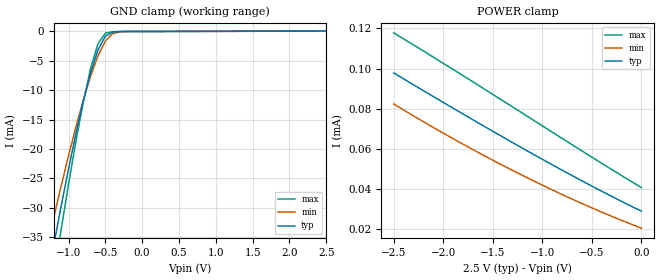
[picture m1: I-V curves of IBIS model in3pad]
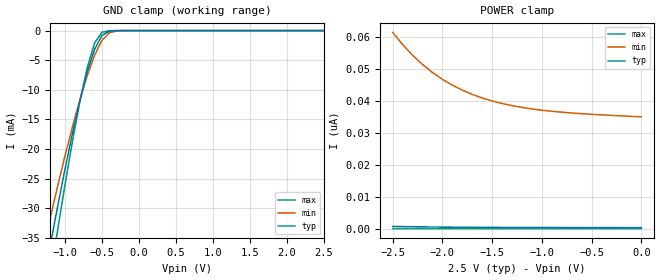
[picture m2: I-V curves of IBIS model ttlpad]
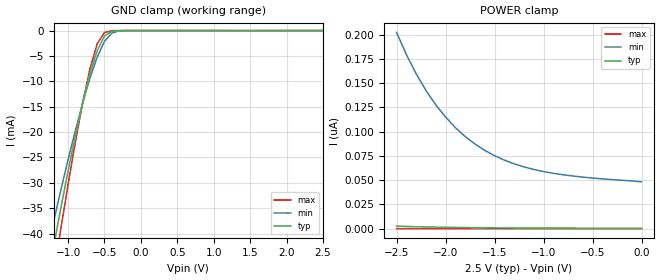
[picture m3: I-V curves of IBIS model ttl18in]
| IBIS file idt45t905z.ibs created by s2ibis2 version 1.2
| North Carolina State University Electronics Research Laboratory  1995
[IBIS ver]   3.2
[File name]   idt45t905z.ibs
[File Rev]   1.0
[Date]   Friday, November 09, 2001
[Source]   Integrated Device Technology, Inc.
[Notes]   Input pins <A> and <AX> can be configured as one of the
   following three models: ttl25in, ttl18in, or hstlin.
   Output pins <Q1> to <Q5> can be configured as one of the
   following three models: ttl25out, ttl18out, or hstlout.
   Please change the column 'model_name' in pin list to select
   the correct model.
[Disclaimer] Integrated Device Technology, Inc. ("IDT") hereby grants the
   user of this IBIS model a non-exclusive, nontransferable
   license to use this IBIS model under the following terms. The
   user is granted this license only to use the IBIS model and is
   not granted rights to sell, copy (except as needed to run the
   IBIS model), rent, lease or sub-license the IBIS model in
   whole or in part, or in modified form to anyone. The User may
   modify the IBIS model to suit its specific applications, but
   rights to derivative works and such modifications shall belong
   to IDT. This IBIS model is provided on an AS IS" basis and IDT
   makes absolutely no warranty with respect to the information
   contained herein. IDT DISCLAIMS AND CUSTOMER WAIVES ALL
   WARRANTIES, EXPRESS AND IMPLIED, INCLUDING WARRANTIES OF
   MERCHANTABILITY AND FITNESS FOR A PARTICULAR PURPOSE. THE
   ENTIRE RISK AS TO QUALITY AND PERFORMANCE IS WITH THE USER
   ACCORDINGLY, IN NO EVENT SHALL IDT BE LIABLE FOR ANY DIRECT OR
   INDIRECT DAMAGES, WHETHER IN CONTRACT OR TORT, INCLUDING ANY
   LOST PROFITS OR OTHER INCIDENTAL, CONSEQUENTIAL, EXEMPLARY, OR
   PUNITIVE DAMAGES ARISING OUT OF THE USE OR APPLICATION OF THE
   IBIS model. Further, IDT reserves the right to make changes
   without notice to any product herein to improve reliability,
   function, or design. IDT does not convey any license under
   patent rights or any other intellectual property rights,
   including those of third parties. IDT is not obligated to
   provide maintenance or support for the licensed IBIS model.
[Copyright]   Copyright 2001, Integrated Device Technology, Inc. all rights
   reserved
|   Component idt45t905z
[Component]   idt45t905z
[Manufacturer]   Integrated Device Technology
|Package   PG28
[Package]
| variable   typ   min   max
R_pkg   2.40000m   2.40000m   2.40000m
L_pkg   0.90000nH   0.90000nH   0.90000nH
C_pkg   60.0000fF   60.0000fF   60.0000fF
[Pin]  signal_name   model_name   R_pin   L_pin   C_pin
1   GL   ttlpad
2   VDD   POWER
3   GND   GND
4   GX   ttlpad
5   VDDQ   POWER
6   Q1   ttl25out
7   AX   ttl25in
8   A   ttl25in
9   Q5   ttl25out
10   VDDQ   POWER
11   GND   GND
12   VDD   POWER
13   VDD   POWER
14   RxS   in3pad
15   TxS   in3pad
16   VDDQ   POWER
17   GND   GND
18   GND   GND
19   VDDQ   POWER
20   Q4   ttl25out
21   Q3   ttl25out
22   GND   GND
23   Q2   ttl25out
24   VDDQ   POWER
25   GND   GND
26   GND   GND
27   VDDQ   POWER
28   GND   GND
[Pin Mapping]  pulldown_ref   pullup_ref   gnd_clamp_ref   power_clamp_ref
1   GND   VDD
2   NC   VDD
3   GND   NC
4   GND   VDD
5   NC   VDDQ
6   GND   VDDQ
7   GND   VDD
8   GND   VDD
9   GND   VDDQ
10   NC   VDDQ
11   GND   NC
12   NC   VDD
13   NC   VDD
14   GND   VDD
15   GND   VDD
16   NC   VDDQ
17   GND   NC
18   GND   NC
19   NC   VDDQ
20   GND   VDDQ
21   GND   VDDQ
22   GND   NC
23   GND   VDDQ
24   NC   VDDQ
25   GND   NC
26   GND   NC
27   NC   VDDQ
28   GND   NC
| Models and submodels in the file (8): in3pad (Input), ttlpad (Input), ttl18in (Input), ttl25in (Input), hstlin (Input), ttl18out (Output), ttl25out (Output), hstlout (Output)
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|   Model in3pad
[Model]   in3pad
Model_type   Input
Polarity   Non-Inverting
Vinl =  0.70000V
Vinh =  1.70000V
Vmeas =  1.25000V
C_comp   5.00000pF   5.00000pF   5.00000pF
[Temperature Range]   45.00000   0.14000k   -30.00000
[Voltage Range]   2.50000V   2.30000V   2.70000V
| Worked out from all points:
|   GND clamp passes 1 mA (typ) near -0.51 V on its own axis
[GND_clamp]
| voltage   I(typ)   I(min)   I(max)
-2.5V     -129.2mA   -109.1mA   -150.7mA
-1.3V     -43.03mA   -37.1mA    -49.76mA
-1.2V     -36.26mA   -31.58mA   -41.61mA
-1.1V     -29.68mA   -26.24mA   -33.65mA
-900mV    -17.38mA   -16.25mA   -18.7mA
-800mV    -11.87mA   -11.72mA   -12.03mA
-700mV    -7.017mA   -7.631mA   -6.282mA
-600mV    -3.163mA   -4.169mA   -2.108mA
-500mV    -846.7uA   -1.655mA   -328.1uA
-400mV    -132.2uA   -398uA     -66.99uA
-300mV    -41.75uA   -74.33uA   -49.92uA
2.5V      28.85uA    24.24uA    34.77uA
[POWER_clamp]
| voltage   I(typ)   I(min)   I(max)
-2.5V     97.81uA    82.34uA    117.8uA
-1.9V     80.2uA     64.99uA    99.56uA
-1.5V     68.7uA     54.27uA    87.12uA
-1.2V     60.25uA    46.68uA    77.7uA
-600mV    43.96uA    32.66uA    58.9uA
-300mV    36.22uA    26.27uA    49.65uA
0V        28.85uA    20.35uA    40.61uA
|   Model ttlpad
[Model]   ttlpad
Model_type   Input
Polarity   Non-Inverting
Vinl =  0.70000V
Vinh =  1.70000V
Vmeas =  1.25000V
C_comp   5.00000pF   5.00000pF   5.00000pF
[Temperature Range]   45.00000   0.14000k   -30.00000
[Voltage Range]   2.50000V   2.30000V   2.70000V
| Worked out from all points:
|   GND clamp passes 1 mA (typ) near -0.51 V on its own axis
[GND_clamp]
| voltage   I(typ)   I(min)   I(max)
-2.5V     -129.2mA   -109.1mA   -150.6mA
-1.3V     -43.01mA   -37.08mA   -49.74mA
-1.2V     -36.24mA   -31.57mA   -41.59mA
-1.1V     -29.66mA   -26.23mA   -33.63mA
-900mV    -17.36mA   -16.23mA   -18.68mA
-800mV    -11.85mA   -11.7mA    -12mA
-700mV    -6.996mA   -7.615mA   -6.253mA
-600mV    -3.137mA   -4.151mA   -2.071mA
-500mV    -815.1uA   -1.634mA   -278.8uA
-400mV    -95.37uA   -373.7uA   -14.75uA
-300mV    -5.658uA   -48.78uA   -281.7nA
2.5V      324.7pA    35.28nA    828.2fA
[POWER_clamp]
| voltage   I(typ)   I(min)   I(max)
-2.5V     698.6pA    61.39nA    2.05pA
-2.4V     644.6pA    57.56nA    1.88pA
-2.3V     597.5pA    54.23nA    1.737pA
-2.2V     556.7pA    51.34nA    1.611pA
-2.1V     521.4pA    48.85nA    1.499pA
-1.9V     465pA      44.88nA    1.333pA
-1.8V     442.7pA    43.32nA    1.256pA
-1.6V     407.7pA    40.88nA    1.155pA
-1.3V     373.1pA    38.48nA    1.037pA
-1V       352.5pA    37.05nA    965.9fA
-600mV    337.2pA    35.97nA    899.5fA
0V        324.7pA    34.99nA    849.9fA
|   Model ttl18in
[Model]   ttl18in
Model_type   Input
Polarity   Non-Inverting
Vinl =  0.68V
Vinh =  1.07V
Vmeas =  0.9V
C_comp   5.00000pF   5.00000pF   5.00000pF
[Temperature Range]   45.00000   0.14000k   -30.00000
[Voltage Range]   2.50000V   2.30000V   2.70000V
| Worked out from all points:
|   GND clamp passes 1 mA (typ) near -0.49 V on its own axis
[GND_clamp]
| voltage   I(typ)   I(min)   I(max)
-2.5V     -150.1mA   -128.5mA   -173mA
-1.3V     -50.47mA   -44.23mA   -57.51mA
-1.2V     -42.64mA   -37.76mA   -48.2mA
-1.1V     -35.02mA   -31.48mA   -39.1mA
-900mV    -20.73mA   -19.68mA   -21.96mA
-800mV    -14.28mA   -14.3mA    -14.26mA
-700mV    -8.553mA   -9.407mA   -7.567mA
-600mV    -3.939mA   -5.223mA   -2.609mA
-500mV    -1.074mA   -2.122mA   -375.8uA
-400mV    -131.3uA   -507.1uA   -20.31uA
-300mV    -7.825uA   -67.79uA   -384.6nA
2.5V      443.6pA    49.9nA     1.135pA
[POWER_clamp]
| voltage   I(typ)   I(min)   I(max)
-2.5V     2.616nA    202.4nA    8.153pA
-2.4V     2.294nA    179.5nA    7.17pA
-2.3V     2.014nA    159.7nA    6.305pA
-2.2V     1.772nA    142.5nA    5.573pA
-2.1V     1.564nA    127.7nA    4.925pA
-1.9V     1.231nA    104.2nA    3.911pA
-1.8V     1.1nA      95.05nA    3.496pA
-1.6V     895.6pA    80.73nA    2.854pA
-1.3V     696.3pA    66.86nA    2.22pA
-1V       581.4pA    58.89nA    1.825pA
-600mV    500.6pA    53.16nA    1.519pA
0V        443.6pA    48.28nA    1.265pA
